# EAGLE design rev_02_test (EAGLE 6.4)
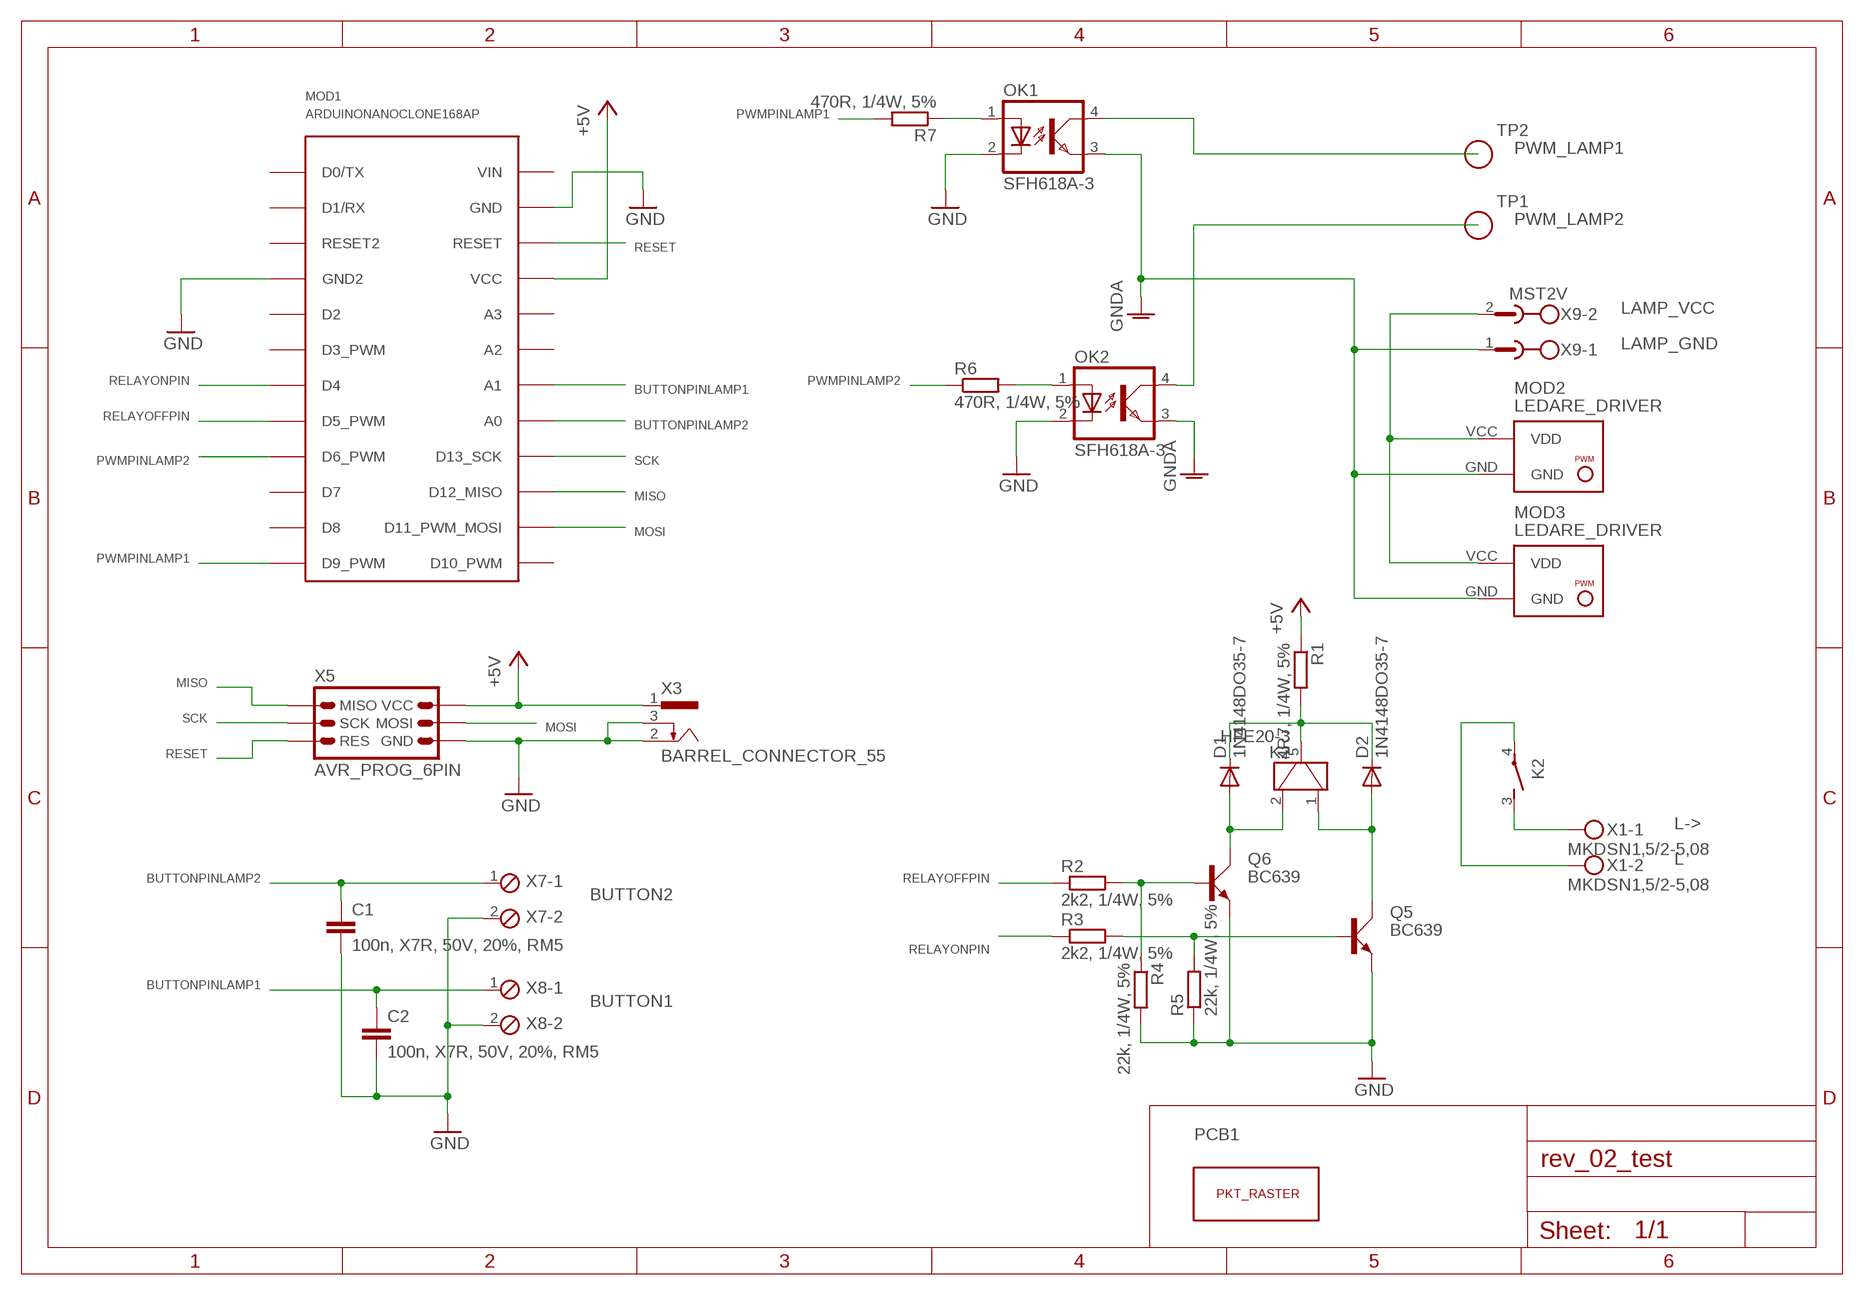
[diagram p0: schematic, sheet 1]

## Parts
C1  100n, X7R, 50V, 20%, RM5  C-EU050-024X044  [C050-024X044]
C2  100n, X7R, 50V, 20%, RM5  C-EU050-024X044  [C050-024X044]
D1  1N4148DO35-7  [DO35-7]
D2  1N4148DO35-7  [DO35-7]
K2  HFE20-3  [HFE20-3]
MOD1  ARDUINONANOCLONE168AP  [ARDUINONANOCLONE]
MOD2  LEDARE_DRIVER  [LEDARE_DRIVER]
MOD3  LEDARE_DRIVER  [LEDARE_DRIVER]
OK1  SFH618A-3  [DIP4]
OK2  SFH618A-3  [DIP4]
PCB1  PUNKTRASTER  [PUNKTRASTER]
Q5  BC639  [SOT54D]
Q6  BC639  [SOT54D]
R1  4R7, 1/4W, 5%  R-EU_0207/12  [0207/12]
R2  2k2, 1/4W, 5%  R-EU_0207/12  [0207/12]
R3  2k2, 1/4W, 5%  R-EU_0207/12  [0207/12]
R4  22k, 1/4W, 5%  R-EU_0207/2V  [0207/2V]
R5  22k, 1/4W, 5%  R-EU_0207/2V  [0207/2V]
R6  470R, 1/4W, 5%  R-EU_0207/2V  [0207/2V]
R7  470R, 1/4W, 5%  R-EU_0207/5V  [0207/5V]
TP1  TP  [TP_THT]
TP2  TP  [TP_THT]
X1  MKDSN1,5/2-5,08  [MKDSN1,5/2-5,08]
X3  BARREL_CONNECTOR_55  [BARREL_CONNECTOR_55]
X5  AVR_PROG_6PIN  [FE03-2]
X7  MPT2  [2POL254]
X8  MPT2  [2POL254]
X9  MST2V  [MSTBV2]

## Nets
+5V: MOD1.VCC R1.1 X3.1 X5.2(VCC)
BUTTONPINLAMP1: C2.1 MOD1.A1 X8.1
BUTTONPINLAMP2: C1.1 MOD1.A0 X7.1
GND: C1.2 C2.2 MOD1.GND MOD1.GND2 OK1.2(C) OK2.2(C) Q5.E Q6.E R4.2 R5.1 X3.2 X3.3 X5.6(GND) X7.2 X8.2
L: K2.4 X1.2
L->: K2.3 X1.1
LAMP_GND: MOD2.GND MOD3.GND OK1.3(EMIT) OK2.3(EMIT) X9.1 ; supply symbol labelled GNDA
LAMP_VCC: MOD2.VCC(VDD) MOD3.VCC(VDD) X9.2
MISO: MOD1.MISO(D12_MISO) X5.1(MISO)
MOSI: MOD1.MOSI(D11_PWM_MOSI) X5.4(MOSI)
N$1: D1.C D2.C K2.5 R1.2
N$2: D2.A K2.1 Q5.C
N$3: D1.A K2.2 Q6.C
N$4: OK2.1(A) R6.2
N$5: Q5.B R3.2 R5.2
N$6: Q6.B R2.2 R4.1
N$7: OK1.1(A) R7.1
PWM_LAMP1: OK1.4(COL) TP2.P$1
PWM_LAMP2: OK2.4(COL) TP1.P$1
PWMPINLAMP1: MOD1.D9(D9_PWM) R7.2
PWMPINLAMP2: MOD1.D6(D6_PWM) R6.1
RELAYOFFPIN: MOD1.D5(D5_PWM) R2.1
RELAYONPIN: MOD1.D4 R3.1
RESET: MOD1.RESET X5.5(RES)
SCK: MOD1.SCK(D13_SCK) X5.3(SCK)
Unconnected: MOD1.A2 MOD1.A3 MOD1.D2 MOD1.D3(D3_PWM) MOD1.D7 MOD1.D8 MOD1.D10(D10_PWM) MOD1.RAW(VIN) MOD1.RESET2 MOD1.RXD(D1/RX) MOD1.TXD(D0/TX)

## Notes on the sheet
- BUTTON2
- BUTTON1

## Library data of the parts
C1 C2 = rcl:C-EU: CAPACITOR, European symbol
D1 D2 = diode:1N4148: DIODE
K2 = my_conns:HFE20-3
MOD1 = my_conns:ARDUINONANOCLONE168AP
MOD2 MOD3 = my_conns:LEDARE_DRIVER
OK1 OK2 = optocoupler:SFH618?*: Optocoupler, Phototransistor Output, Low Input Current Source: Data sheet; MF: VISHAY/TELEFUNKEN; MPN: SFH618A-3; OC_FARNELL: 1020374; OC_NEWARK: 58K2209
PCB1 = my_conns:PUNKTRASTER
Q5 Q6 = transistor-small-signal:BC639: NPN TRANSISTOR
R1-R3 R7 = rcl:R-EU_: RESISTOR, European symbol; OC_REICHELT: 1/4W; PART_VALUE: 1/4W 5%
R4-R6 = rcl:R-EU_: RESISTOR, European symbol
TP1 TP2 = my_conns:TP
X1 = con-phoenix-508:MKDSN1,5/2-5,08: MKDSN 1,5/ 2-5,08 Printklemme; MPN: MKDSN 1,5/2-5.08; OC_FARNELL: 1792903; OC_NEWARK: 30M2397
X3 = my_conns:BARREL_CONNECTOR_55
X5 = my_conns:AVR_PROG_6PIN: AVR ISP prgrammer interface 6 pin
X7 X8 = con-phoenix-254:MPT2: PHOENIX CONNECTOR; OC_FARNELL: unknown; OC_NEWARK: unknown
X9 = con-phoenix-508:MST2V: PHOENIX; OC_FARNELL: unknown; OC_NEWARK: unknown

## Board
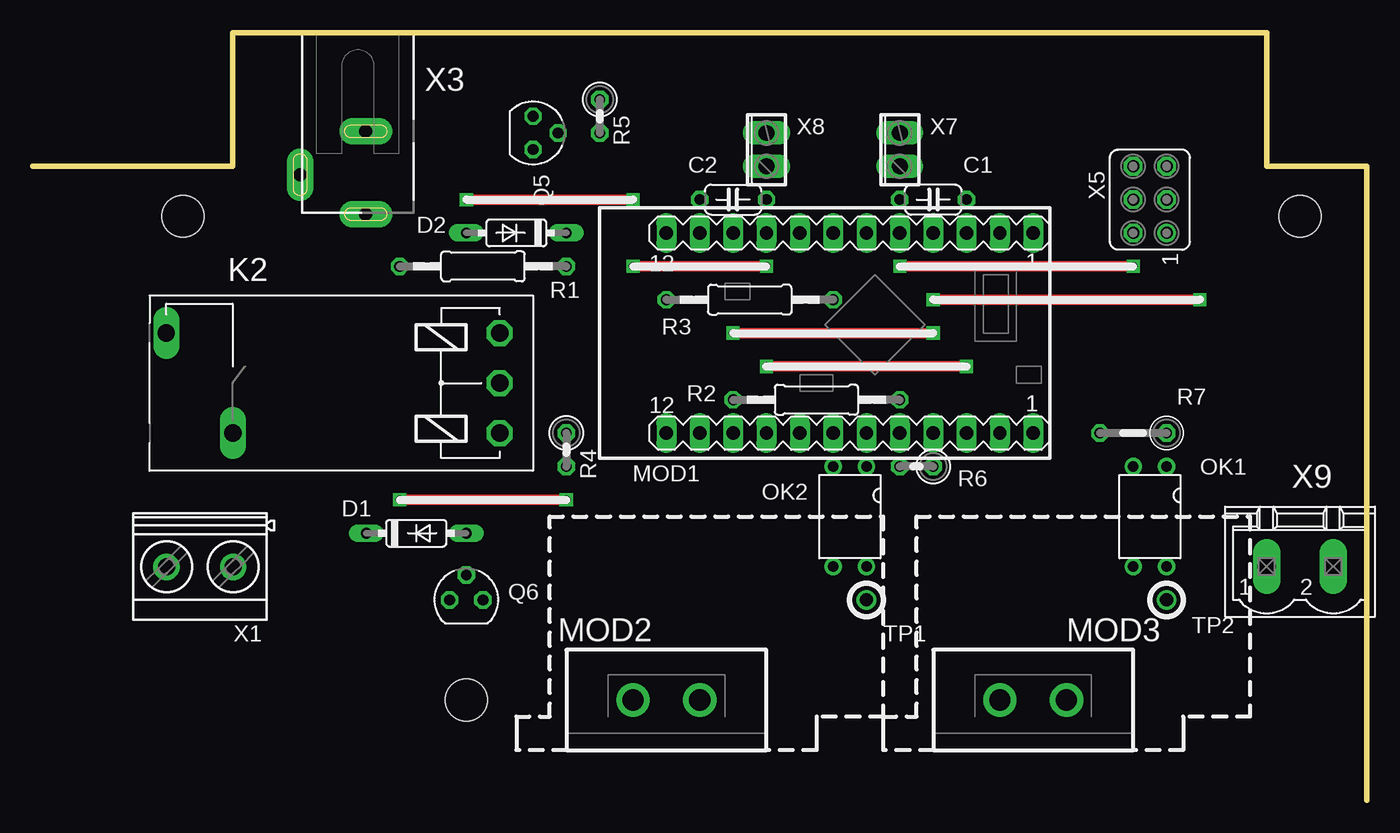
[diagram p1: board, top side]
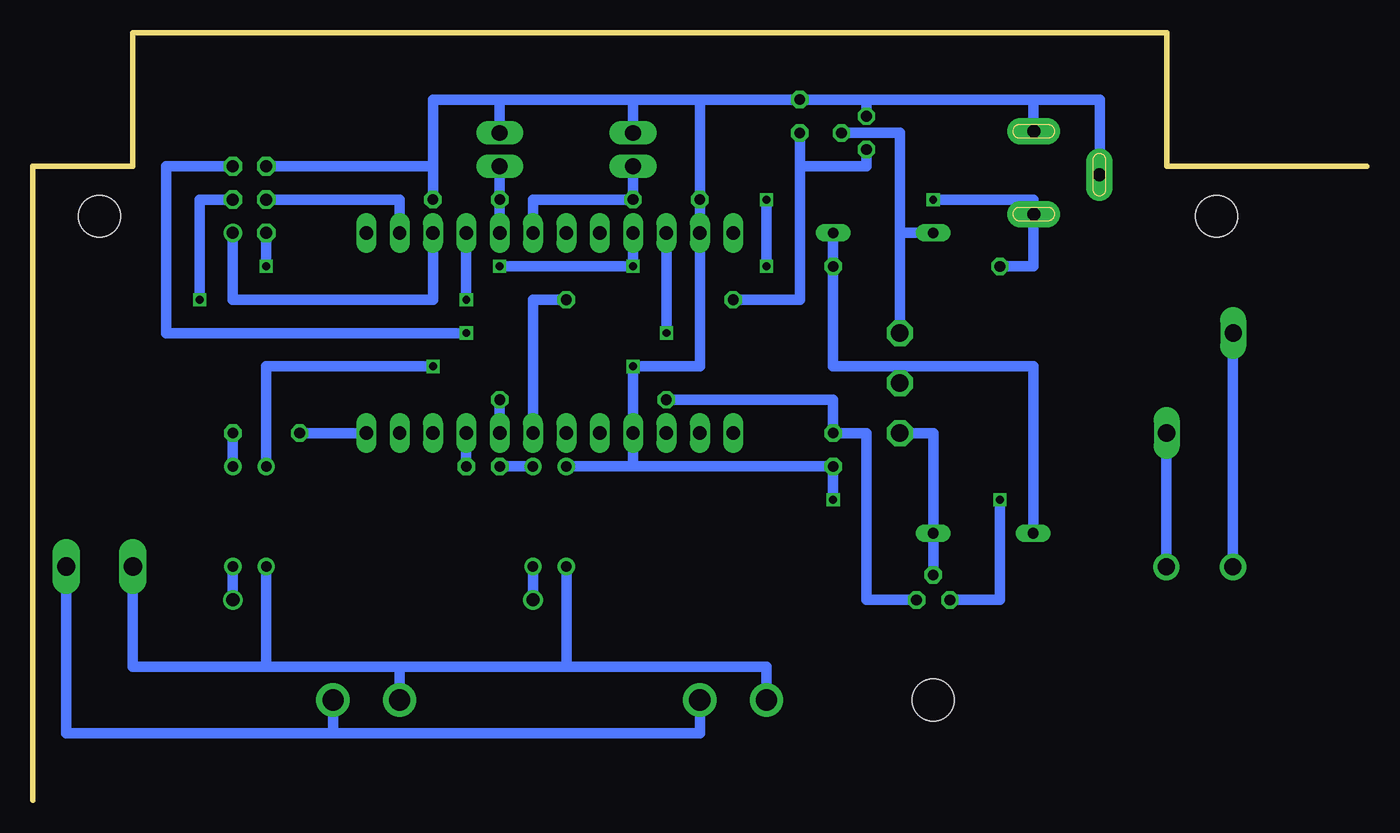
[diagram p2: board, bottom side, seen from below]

Size 101.6 x 58.42 mm. Coordinates in mm from the lower left corner, seen from the top.
Outline: 101.6,0 101.6,48.26 93.98,48.26 93.98,58.42 15.24,58.42 15.24,48.26 0,48.26
Copper layers (1*16): Top 0.035mm / dielectric 1.5mm / Bottom 0.035mm
Design rules "default": minimum track width 10mil, minimum drill 24mil, track to track 8mil, track to pad 8mil, pad to pad 8mil, via to via 8mil, smd to smd 8mil, copper to edge 40mil, drill to drill 8mil, minimum pad ring 10mil, minimum via ring 8mil, stop-mask expansion 4mil, vias tented up to drill 0mil, thermal gap 10mil
Holes 3.2 mm at 11.43,44.45 96.52,44.45 33.02,7.62
vRestrict: area 92.7,40.6 to 100.3,48.3; area 7.6,40.6 to 15.2,48.3; area 29.2,3.8 to 36.8,11.4; 10 lines

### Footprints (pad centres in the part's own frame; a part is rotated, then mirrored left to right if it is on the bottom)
C050-024X044 = drill 0.813 octagon: 1 -2.54,0; 2 2.54,0
DO35-7 = drill 0.813 long: A 3.81,0; C -3.81,0
HFE20-3 = drill 1.321 octagon: 1 -11.43,-3.81; 2 -11.43,3.81; 5 -11.43,0 | drill 1.321 long: 3 8.89,3.81; 4 13.97,-3.81
ARDUINONANOCLONE = drill 1.016 long: A0 17.78,0; A1 15.24,0; A2 12.7,0; A3 10.16,0; D2 10.16,-15.24; D3 12.7,-15.24; D4 15.24,-15.24; D5 17.78,-15.24; D6 20.32,-15.24; D7 22.86,-15.24; D8 25.4,-15.24; D9 27.94,-15.24; D10 27.94,0; GND 2.54,0; GND2 7.62,-15.24; MISO 22.86,0; MOSI 25.4,0; RAW 0,0; RESET 5.08,0; RESET2 5.08,-15.24; RXD 2.54,-15.24; SCK 20.32,0; TXD 0,-15.24; VCC 7.62,0
LEDARE_DRIVER = drill 1.6 pad 2.54: GND 0,0; VCC 5.08,0
DIP4 = drill 0.8: 1 -1.27,-3.81; 2 1.27,-3.81; 3 1.27,3.81; 4 -1.27,3.81
SOT54D = drill 0.813 octagon: B 1.27,0; C 0,1.905; E -1.27,0
0207/12 = drill 0.813 octagon: 1 -6.35,0; 2 6.35,0
0207/2V = drill 0.813 octagon: 1 -1.27,0; 2 1.27,0
0207/5V = drill 0.813 octagon: 1 -2.54,0; 2 2.54,0
TP_THT = drill 1 pad 1.422: P$1 0,0
MKDSN1,5/2-5,08 = drill 1.3 pad 2: 1 -2.561,0.025; 2 2.519,0.025
BARREL_CONNECTOR_55 = drill 1 pad 2 long: 1 -2.5,13.8; 2 -2.5,7.5; 3 2.5,10.8
FE03-2 = drill 0.914: 1 0,-2.54 | drill 0.914 octagon: 2 0,0; 3 2.54,-2.54; 4 2.54,0; 5 5.08,-2.54; 6 5.08,0
2POL254 = drill 1.2 long: 1 -1.27,0; 2 1.27,0
MSTBV2 = drill 1.397 long: 1 -2.54,0; 2 2.54,0

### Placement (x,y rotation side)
C1  68.58,45.72 0 top
C2  53.34,45.72 180 top
D1  29.21,20.32 0 top
D2  36.83,43.18 180 top
K2  24.13,31.75 180 top
MOD1  48.26,43.18 0 top
MOD2  45.72,7.62 0 top
MOD3  73.66,7.62 0 top
OK1  85.09,21.59 180 top
OK2  62.23,21.59 180 top
PCB1  10.16,7.62 0 top
Q5  38.1,50.8 270 top
Q6  33.02,15.24 0 top
R1  34.29,40.64 0 top
R2  59.69,30.48 180 top
R3  54.61,38.1 180 top
R4  40.64,26.67 270 top
R5  43.18,52.07 270 top
R6  67.31,25.4 180 top
R7  83.82,27.94 180 top
TP1  63.5,15.24 0 top
TP2  86.36,15.24 0 top
X1  12.7,17.78 180 top
X3  22.86,58.42 180 top
X5  83.82,43.18 90 top
X7  66.04,49.53 90 top
X8  55.88,49.53 90 top
X9  96.52,17.78 0 top

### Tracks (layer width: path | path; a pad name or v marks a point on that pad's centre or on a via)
+5V  (via drill 0.6)
  Top 0.813: v83.82,40.64 v66.04,40.64 | v33.02,45.72 v45.72,45.72 | v45.72,40.64 v55.88,40.64
  Bottom 0.813: X5.2 v83.82,40.64 | v33.02,45.72 25.4,45.72 25.4,44.62 | v45.72,45.72 v45.72,40.64 | MOD1.VCC v55.88,40.64 v66.04,40.64 | X3.1 25.4,44.62 | 25.4,44.62 25.4,40.64 R1.1
BUTTONPINLAMP1
  Bottom 0.813: X8.1 C2.1 63.5,45.72 MOD1.A1
BUTTONPINLAMP2
  Bottom 0.813: MOD1.A0 C1.1 X7.1
GND  (via drill 0.6)
  Top 0.813: v27.94,22.86 v40.64,22.86 | v71.12,33.02 v55.88,33.02
  Bottom 0.813: 55.88,53.34 66.04,53.34 | X7.2 66.04,53.34 | 66.04,53.34 71.12,53.34 | 71.12,53.34 71.1,48.26 X5.6 | 50.8,53.34 R5.1 38.1,53.34 | 55.88,25.4 R4.2 v40.64,22.86 | 50.8,53.34 C2.2 MOD1.GND 50.8,33.02 v55.88,33.02 MOD1.GND2 55.88,25.4 | 55.88,25.4 OK2.2 | 50.8,53.34 55.88,53.34 | 55.88,53.34 X8.2 | C1.2 71.12,53.34 | OK1.2 83.82,33.02 v71.12,33.02 | 25.4,53.34 25.4,50.92 X3.2 | 25.4,53.34 20.32,53.34 20.32,47.62 X3.3 | 25.4,53.34 38.1,53.34 | Q5.E 38.1,53.34 | Q6.E 27.94,15.24 v27.94,22.86
L
  Bottom 0.813: K2.4 10.18,33.02 X1.2
L->
  Bottom 0.813: 15.24,17.78 15.26,17.78 X1.1 15.26,25.4 K2.3
LAMP_GND
  Bottom 0.813: 73.66,10.16 83.82,10.16 | 83.82,10.16 93.98,10.16 X9.1 | MOD3.GND 73.66,10.16 | 73.66,10.16 60.96,10.16 | 60.96,10.16 45.72,10.16 MOD2.GND | OK2.3 60.96,10.16 | OK1.3 83.82,10.16
LAMP_VCC
  Bottom 0.813: X9.2 99.06,5.08 78.74,5.08 | MOD3.VCC 78.74,5.08 | MOD2.VCC 50.8,5.08 78.74,5.08
MISO
  Bottom 0.813: MOD1.MISO 71.12,38.1 86.36,38.1 X5.1
MOSI
  Bottom 0.813: MOD1.MOSI 73.66,45.72 X5.4
N$1
  Bottom 0.813: D2.C R1.2 40.64,33.02 35.56,33.02 | D1.C 25.4,33.02 35.56,33.02 | K2.5 35.56,33.02
N$2
  Bottom 0.813: 35.56,43.18 35.56,50.8 Q5.C | K2.1 35.56,43.18 | 35.56,43.18 D2.A
N$3
  Bottom 0.813: K2.2 33.02,27.94 D1.A Q6.C
N$4
  Bottom 0.813: OK2.1 R6.2
N$5
  Bottom 0.813: R5.2 43.18,48.26 | 43.18,48.26 43.18,38.1 R3.2 | Q5.B 38.1,48.26 43.18,48.26
N$6
  Bottom 0.813: R2.2 40.64,30.48 R4.1 38.1,27.94 38.1,15.24 Q6.B
N$7
  Bottom 0.813: R7.1 OK1.1
PWM_LAMP1
  Bottom 0.813: TP2.P$1 OK1.4
PWM_LAMP2
  Bottom 0.813: TP1.P$1 OK2.4
PWMPINLAMP1
  Bottom 0.813: MOD1.D9 R7.2
PWMPINLAMP2
  Bottom 0.813: MOD1.D6 R6.1
RELAYOFFPIN
  Bottom 0.813: R2.1 MOD1.D5
RELAYONPIN
  Bottom 0.813: MOD1.D4 63.5,38.1 R3.1
RESET  (via drill 0.6)
  Top 0.813: v53.34,35.56 v68.58,35.56
  Bottom 0.813: MOD1.RESET v53.34,35.56 | X5.5 91.44,48.26 91.44,35.56 v68.58,35.56
SCK  (via drill 0.6)
  Top 0.813: v68.58,38.1 v88.9,38.1
  Bottom 0.813: MOD1.SCK v68.58,38.1 | X5.3 88.9,45.72 v88.9,38.1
